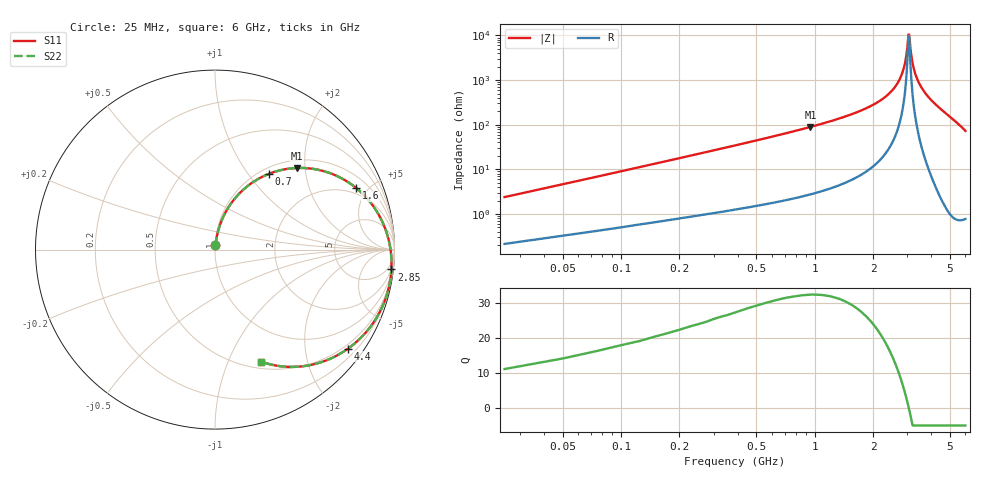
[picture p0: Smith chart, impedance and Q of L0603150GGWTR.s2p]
!	AVX Thin Film Operation
!	Date:	March	2003
!	Description: Accu-L® Series Thin Film SMD RF Inductors
!	Part Number: L0603150GGWTR
!	25MHz-6GHz
!	Serial	Measurements
#	mhz	S	db	R	50
!	S11	S11	S21	S21	S12	S12	S22	S22
!	dB	Phase	dB	Phase	dB	Phase	dB	Phase
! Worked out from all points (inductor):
!   240 points, 25 MHz to 6 GHz, reference 50 ohm
!   read as one part in series: L = 14.5 nH near 50 MHz
!   highest Q = 32.5 at 950 MHz (marker M1), where L = 15 nH
!   self-resonance near 3.05 GHz
!   S11 on the Smith chart (normalised r, x): 25 MHz: 1.00, +0.05; 700 MHz: 1.10, +1.26; 1.6 GHz: 1.61, +4.22; 2.85 GHz: 2, -18; 4.4 GHz: 0.39, -2.98; 6 GHz: 0.58, -1.32
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25  -32.71 83.4  -0.02 -1.4  -0.02 -1.4  -32.71 83.4
75  -23.61 82.3  -0.06 -4.0  -0.06 -4.0  -23.61 82.3
200  -15.46 77.0  -0.19 -10.4  -0.19 -10.4  -15.46 77.0
400  -9.87 67.8  -0.58 -20.0  -0.58 -20.0  -9.87 67.8
700  -5.74 54.7  -1.51 -33.4  -1.51 -33.4  -5.74 54.7
950  -3.81 44.8  -2.55 -43.3  -2.55 -43.3  -3.81 44.8
1025  -3.37 42.1  -2.91 -46.1  -2.91 -46.1  -3.37 42.1
1600  -1.32 23.5  -6.25 -64.4  -6.25 -64.4  -1.32 23.5
2025  -0.61 12.2  -9.62 -75.3  -9.62 -75.3  -0.61 12.2
2550  -0.19 -0.0  -16.18 -85.9  -16.18 -85.9  -0.19 -0.0
2850  -0.10 -6.4  -23.98 -87.6  -23.98 -87.6  -0.10 -6.4
2950  -0.08 -8.5  -29.38 -82.8  -29.38 -82.8  -0.08 -8.5
3025  -0.08 -10.0  -37.18 -60.5  -37.18 -60.5  -0.08 -10.0
3050  -0.08 -10.5  -40.60 -31.8  -40.60 -31.8  -0.08 -10.5
3075  -0.07 -11.0  -40.53 13.3  -40.53 13.3  -0.07 -11.0
3125  -0.08 -12.0  -33.93 53.5  -33.93 53.5  -0.08 -12.0
3200  -0.08 -13.5  -27.84 65.1  -27.84 65.1  -0.08 -13.5
3400  -0.11 -17.5  -20.33 68.3  -20.33 68.3  -0.11 -17.5
4025  -0.39 -29.5  -11.58 59.5  -11.58 59.5  -0.39 -29.5
4400  -0.68 -36.6  -8.90 52.9  -8.90 52.9  -0.68 -36.6
5025  -1.43 -48.5  -5.84 41.3  -5.84 41.3  -1.43 -48.5
6000  -3.43 -67.7  -2.84 22.4  -2.84 22.4  -3.43 -67.7
